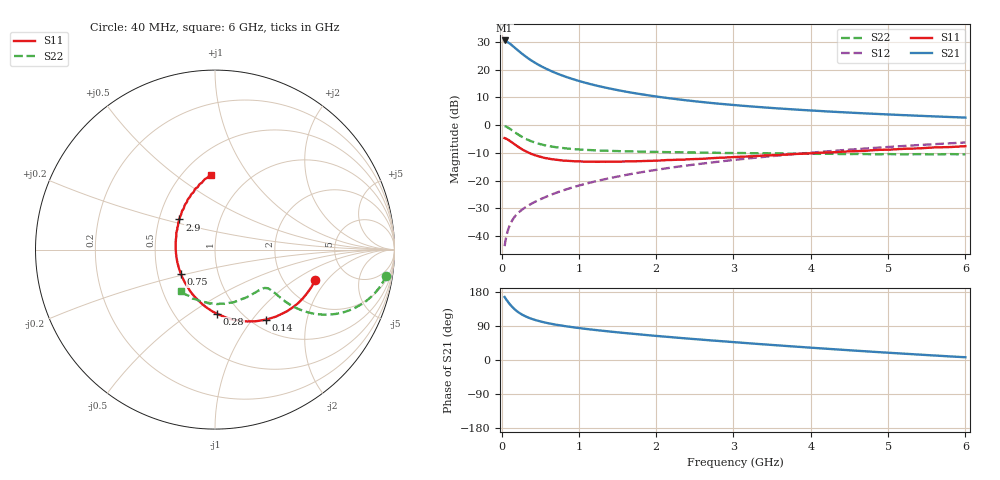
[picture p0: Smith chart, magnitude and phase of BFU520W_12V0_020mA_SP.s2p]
! Filename:  P:\Prog\Test\Noise\ATS_data\Testdata_Net\Run2\BFU520W_APM2013_06_A05_12p0V_020mA_SP_CM01_D.s2p
! Date/Time: Tue 26/Mar/2013 18:01:44
! BFU520W_APM2013_06_A05_12p0V_1to20mA_SP_CM01_Bias8_R.s2p
! MDIF S-parameter v. bias file
! BFU520W_APM2013_06_A05_12p0V_1to20mA_SP_CM01
! Date/time Thu Mar 21 16:35:01 2013
! VAR V_out= 12.0000
! VAR I_out= 19.9950
! VAR V_in= 0.7839
! VAR I_in= 0.2052
! Device data file deembeded for feedlines and parallel
! Original file: \Run2\BFU520W_APM2013_06_A05_12p0V_020mA_SP_CM01_R.s2p
! Feed-files: PR019V01_070313_Feed1.s2p, PR019V01_070313_Feed2.s2p
! Parallel-file: PR019V01_070313_Par.s2p
# MHz S MA R 50
!  Freq-MHz  S11-mag  S11-arg  S21-mag  S21-arg  S12-mag  S12-arg  S22-mag  S22-arg
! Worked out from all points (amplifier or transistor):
!   98 points, 40 MHz to 6 GHz, reference 50 ohm
!   highest |S21| = 30.6 dB at 40 MHz (marker M1)
!   |S21| within 3 dB of that: start of sweep to 187.5 MHz
!   unconditionally stable (mu >= 1): 1.187 GHz to 2.372 GHz
!   at 300 MHz: K = 0.67, MSG = 27.4 dB, |S12| = -29.8 dB
!   at 1.6 GHz: K = 1.01, MAG = 14.4 dB, |S12| = -18.0 dB
!   at 6 GHz: K = 0.88, MSG = 4.5 dB, |S12| = -6.3 dB
!   S11 on the Smith chart (normalised r, x): 40 MHz: 2.95, -1.52; 140 MHz: 1.16, -1.18; 280 MHz: 0.79, -0.64; 750 MHz: 0.66, -0.19; 2.9 GHz: 0.64, +0.23; 6 GHz: 0.67, +0.68
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40  0.5839 -16.9  33.79 166.3  0.006533 81.8  0.9628 -8.7
50  0.5767 -21.1  33.6 163.2  0.007976 80.7  0.9529 -11.0
60  0.5682 -25.2  32.68 160.1  0.00948 79.1  0.9393 -13.1
90  0.5395 -36.8  30.82 151.7  0.01356 75.4  0.8911 -18.7
120  0.5054 -47.5  28.78 144.2  0.01716 72.3  0.8372 -23.3
140  0.4831 -53.9  27.28 139.8  0.01926 70.8  0.8002 -25.8
160  0.4608 -59.9  25.8 135.8  0.0213 69.5  0.7653 -27.9
200  0.4203 -70.6  23.11 128.8  0.02479 67.8  0.7002 -31.1
240  0.3858 -80.1  20.79 123.0  0.02791 67.0  0.6453 -33.3
280  0.3568 -88.4  18.76 118.3  0.0308 66.6  0.599 -34.7
360  0.3142 -102.4  15.56 110.9  0.03631 66.8  0.5295 -36.1
460  0.2794 -116.3  12.71 104.2  0.04305 67.8  0.4718 -36.4
600  0.2503 -131.6  10.08 97.2  0.0526 69.2  0.422 -36.0
750  0.2337 -144.3  8.217 91.7  0.06306 70.2  0.3922 -35.8
1050  0.2203 -163.3  6.002 83.1  0.0846 71.2  0.3607 -36.6
1500  0.2193 176.8  4.293 73.0  0.1179 70.8  0.3402 -40.3
2050  0.2296 159.6  3.217 62.7  0.1595 68.7  0.3282 -47.0
2900  0.2602 139.7  2.378 48.8  0.2267 63.9  0.3138 -60.8
3100  0.2692 135.6  2.249 45.7  0.243 62.5  0.3139 -64.2
4100  0.3161 119.0  1.807 31.1  0.3268 54.9  0.3028 -84.3
5200  0.3735 103.5  1.516 16.7  0.4204 45.2  0.2967 -109.3
6000  0.4174 93.4  1.369 7.2  0.4859 37.5  0.297 -129.8
